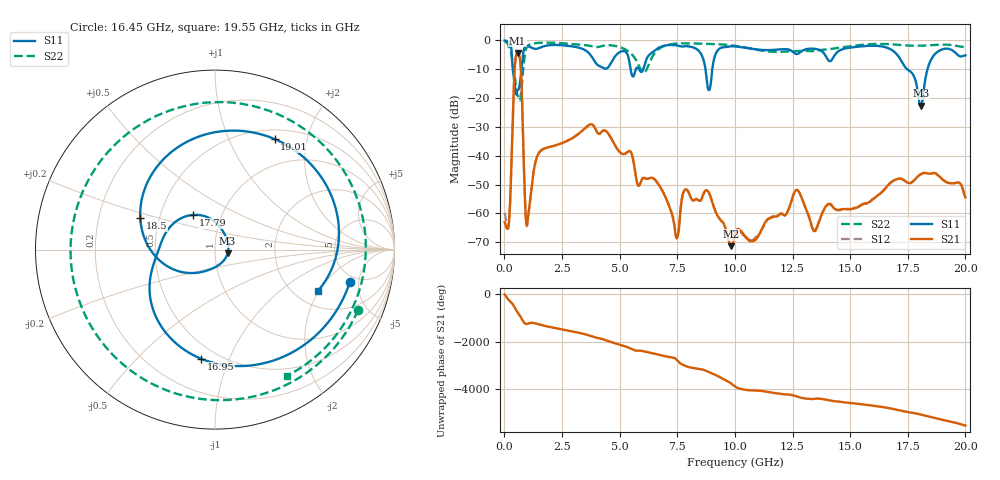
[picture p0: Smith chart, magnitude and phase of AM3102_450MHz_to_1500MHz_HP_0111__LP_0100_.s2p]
!Agilent Technologies,E8364B,MY43040894,A.07.50.67
!Agilent E8364B: A.07.50.67
!Date: Thursday, January 11, 2018 05:51:59
!Correction: S11(Full 2 Port(1,2))
!S21(Full 2 Port(1,2))
!S12(Full 2 Port(1,2))
!S22(Full 2 Port(1,2))
!S2P File: Measurements: S11, S21, S12, S22:
# Hz S  dB  R 50
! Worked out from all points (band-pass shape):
!   1601 points, 10 MHz to 20 GHz, reference 50 ohm
!   highest |S21| = -4.42 dB at 572.2 MHz (marker M1); lowest = -71.4 dB at 9.83 GHz (marker M2)
!   |S21| within 3 dB of the highest: 470.3 MHz to 689 MHz (218.7 MHz wide, 37.7 % of centre)
!   lowest |S11| = -22.7 dB at 18.06 GHz (marker M3), VSWR 1.16, Z = 57.5 - j2.5 ohm
!   |S11| at or under -10 dB: 365.7 MHz to 741.5 MHz (375.8 MHz wide, 67.9 % of centre); 8.724 GHz to 9.02 GHz (296.4 MHz wide, 3.34 % of centre); 17.47 GHz to 18.36 GHz (890.1 MHz wide, 4.97 % of centre)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
!   |S22| runs from -20.8 to -0.3 dB; largest |S21 - S12| = 0.0019
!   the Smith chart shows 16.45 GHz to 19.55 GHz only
!   S11 on the Smith chart (normalised r, x): 16.45 GHz: 4.32, -3.82; 16.95 GHz: 0.41, -0.79; 17.79 GHz: 0.73, +0.30; 18.5 GHz: 0.39, +0.17; 19.01 GHz: 0.62, +1.49; 19.55 GHz: 2.62, -1.95
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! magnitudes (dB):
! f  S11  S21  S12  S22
! 10 MHz  -0.1  -63.1  -59.7  -0.3
! 197.4 MHz  -0.7  -63.1  -63.9  -2.5
! 572.2 MHz  -17.2  -4.4  -4.4  -19.0
! 997 MHz  -2.0  -63.3  -63.7  -2.1
! 1.509 GHz  -2.7  -38.9  -38.9  -0.9
! 3.346 GHz  -2.8  -31.5  -31.5  -1.5
! 6.682 GHz  -2.6  -49.9  -49.9  -3.1
! 7.481 GHz  -1.8  -68.6  -67.6  -1.1
! 8.881 GHz  -17.3  -53.0  -52.9  -1.2
! 9.83 GHz  -2.1  -71.4  -70.8  -1.7
! 10.01 GHz  -2.1  -67.2  -67.5  -1.9
! 12.68 GHz  -4.8  -51.9  -51.8  -3.7
! 13.34 GHz  -2.9  -64.7  -64.6  -3.8
! 16.45 GHz  -2.2  -52.0  -52.1  -1.3
! 16.68 GHz  -2.8  -50.0  -50.0  -1.3
! 16.95 GHz  -4.3  -48.4  -48.4  -1.5
! 17.79 GHz  -12.9  -48.4  -48.4  -1.9
! 18.06 GHz  -22.7  -46.4  -46.5  -1.9
! 18.5 GHz  -6.9  -46.2  -46.3  -1.7
! 19.01 GHz  -3.1  -48.3  -48.2  -1.5
! 19.55 GHz  -4.2  -49.5  -49.5  -1.8
! 20 GHz  -5.2  -54.4  -54.4  -2.5
